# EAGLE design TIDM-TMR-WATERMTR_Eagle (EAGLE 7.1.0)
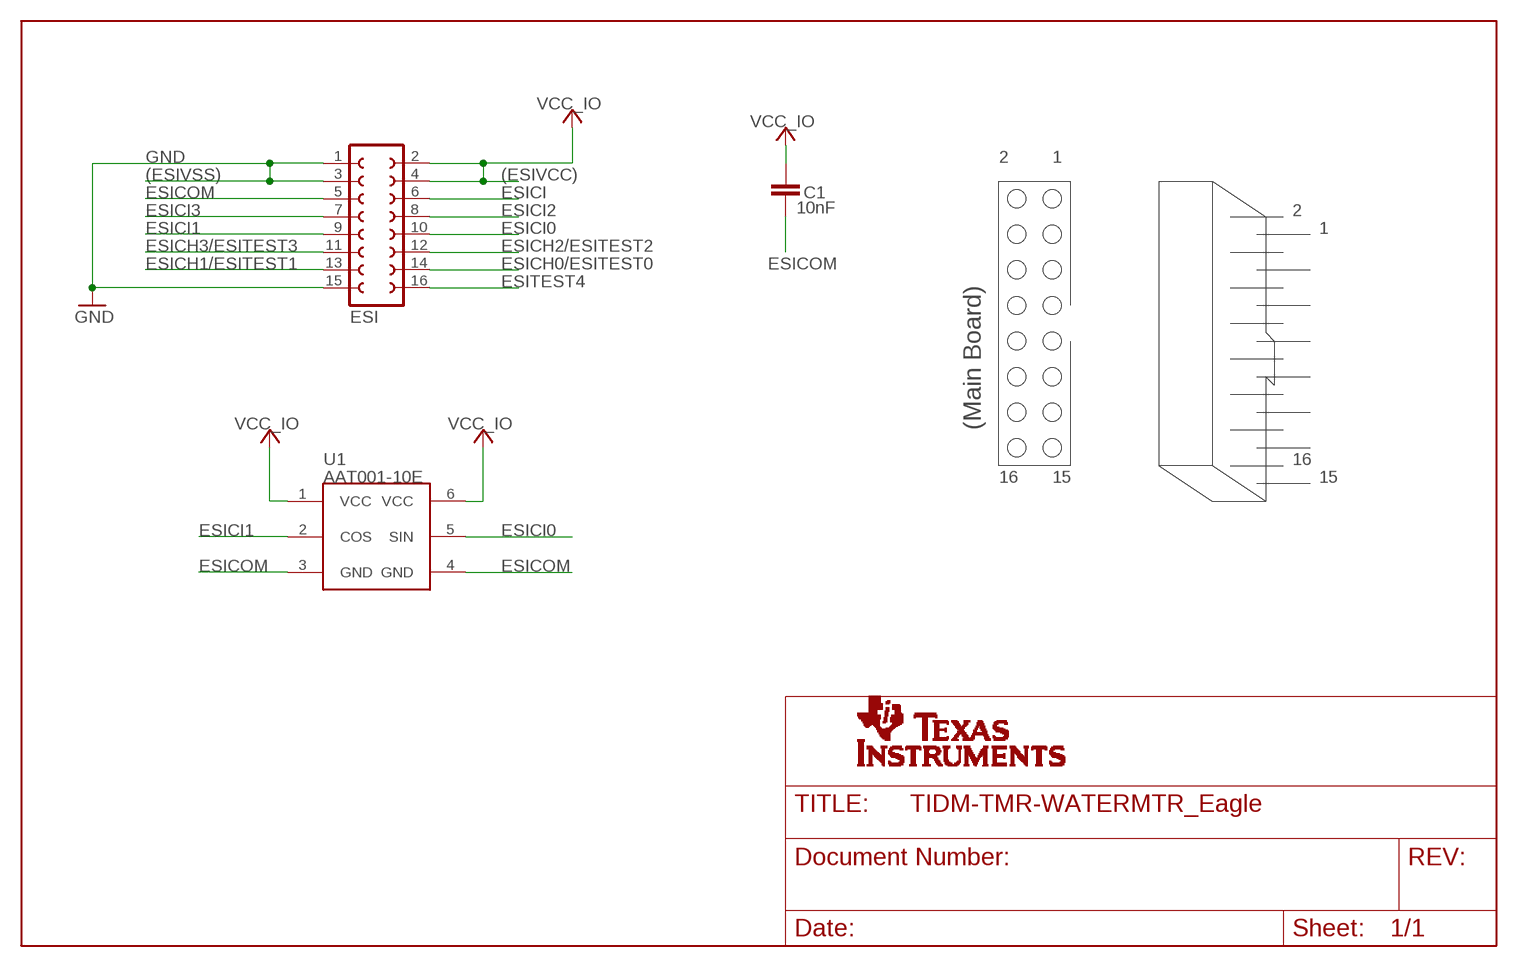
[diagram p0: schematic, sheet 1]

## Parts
C1  10nF  C-EUC0402K  [C0402K]
ESI  FE08-2  [FE08-2]
U1  AAT001-10E  [TDFN6-2.5X2.5MM]
U$1  TI-LOGO-SMALL  [TI-LOGO-4]

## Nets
ESICH0/ESITEST0: ESI.14
ESICH1/ESITEST1: ESI.13
ESICH2/ESITEST2: ESI.12
ESICH3/ESITEST3: ESI.11
ESICI: ESI.6
ESICI0: ESI.10 U1.5(SIN)
ESICI1: ESI.9 U1.2(COS)
ESICI2: ESI.8
ESICI3: ESI.7
ESICOM: C1.2 ESI.5 U1.3(GND) U1.4(GND)
ESITEST4: ESI.16
GND: ESI.1 ESI.3 ESI.15
VCC_IO: C1.1 ESI.2 ESI.4 U1.1(VCC) U1.6(VCC)

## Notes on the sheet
- 2 | 1
- (ESIVSS) | (ESIVCC)
- 2
- 1
- (Main Board)
- 16
- 16 | 15 | 15

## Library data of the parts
C1 = rcl:C-EU: CAPACITOR, European symbol
ESI = con-lsta:FE08-2: FEMALE HEADER; OC_FARNELL: unknown; OC_NEWARK: unknown
U1 = GMR Sensor:AAT001-10E
U$1 = texas-logo:TI-LOGO: Full TI logo

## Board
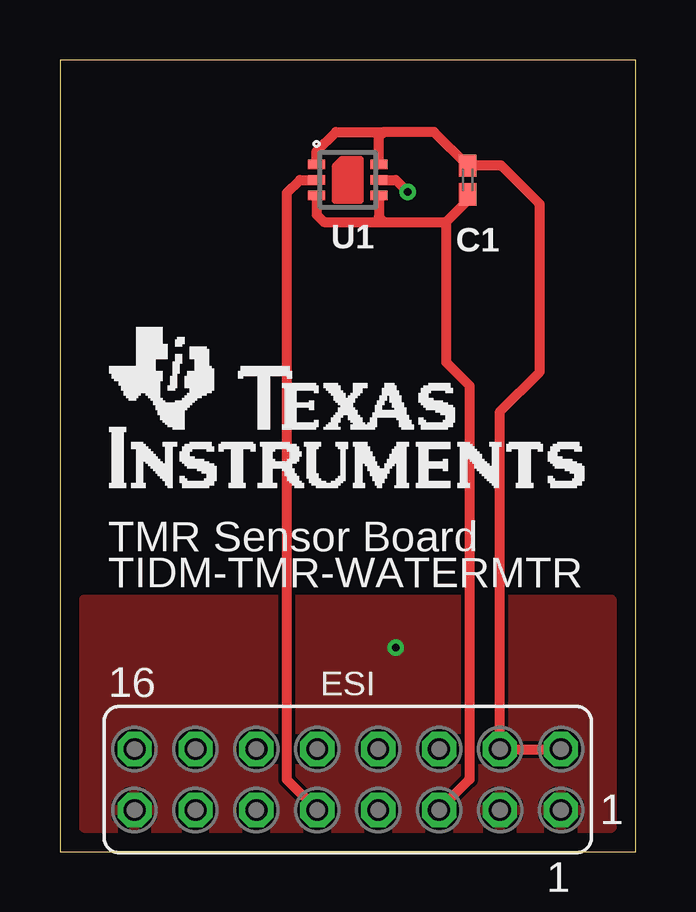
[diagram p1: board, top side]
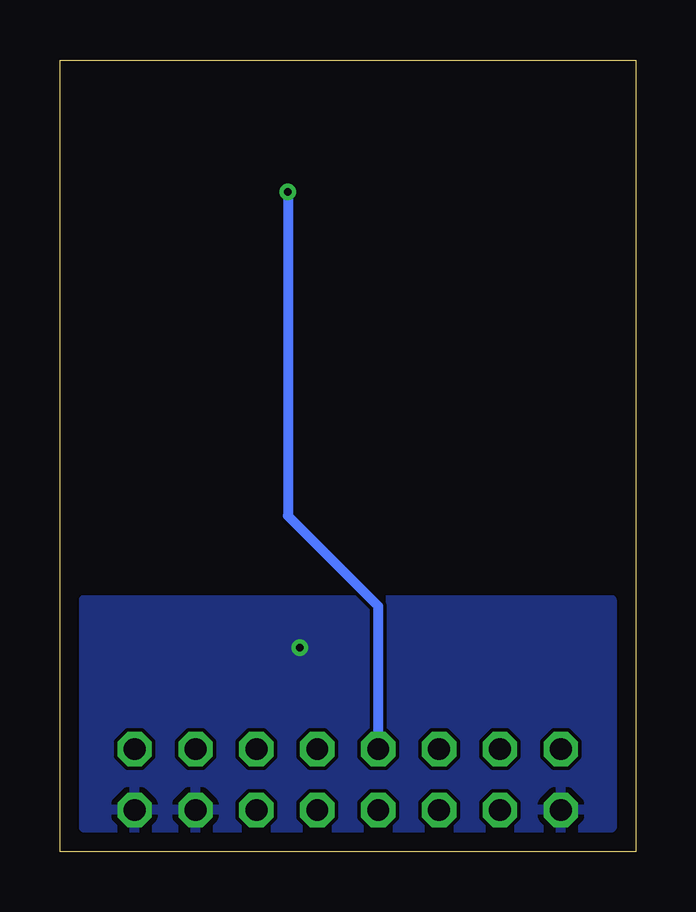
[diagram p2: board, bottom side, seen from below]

Size 24 x 33 mm. Coordinates in mm from the lower left corner, seen from the top.
Outline: 24,0 24,33 0,33 0,0 24,0
Copper layers (1*16): Top 0.035mm / dielectric 1.5mm / Bottom 0.035mm
Design rules "default *": minimum track width 10mil, minimum drill 0.3mm, track to track 6mil, track to pad 6mil, pad to pad 6mil, via to via 6mil, smd to smd 6mil, copper to edge 20mil, drill to drill 8mil, minimum pad ring 10mil, minimum via ring 8mil, stop-mask expansion 4mil, vias tented up to drill 100mil, thermal gap 10mil

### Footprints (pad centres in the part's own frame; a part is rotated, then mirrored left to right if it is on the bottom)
C0402K = smd 0.925 x 0.74: 1 -0.6,0; 2 0.6,0
FE08-2 = drill 0.914 octagon: 1 -8.89,1.27; 2 -8.89,-1.27; 3 -6.35,1.27; 4 -6.35,-1.27; 5 -3.81,1.27; 6 -3.81,-1.27; 7 -1.27,1.27; 8 -1.27,-1.27; 9 1.27,1.27; 10 1.27,-1.27; 11 3.81,1.27; 12 3.81,-1.27; 13 6.35,1.27; 14 6.35,-1.27; 15 8.89,1.27; 16 8.89,-1.27
TDFN6-2.5X2.5MM = smd 0.7 x 0.4: 1 -1.3,0.65; 2 -1.3,0; 3 -1.3,-0.65; 4 1.3,-0.65; 5 1.3,0; 6 1.3,0.65

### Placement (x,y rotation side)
C1  17,28 270 top
ESI  12,3 180 top
U1  12,28 0 top
U$1  2,15 0 top

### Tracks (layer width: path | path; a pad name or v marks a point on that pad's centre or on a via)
ESICI0  (via drill 0.3)
  Top 0.406: U1.5 14,28 v14.5,27.5
  Bottom 0.406: v14.5,27.5 14.5,14 10.73,10.23 ESI.10
ESICI1
  Top 0.406: ESI.9 9.46,3 9.46,27.46 10,28 U1.2
ESICOM
  Top 0.406: U1.3 10.7,26.55 11,26.25 13.5,26.25 | 13.5,26.25 16.1,26.25 | U1.4 13.3,26.45 13.5,26.25 | 16.1,26.25 16.1,20.4 17.08,19.42 17.08,3 ESI.5 | 16.1,26.25 17,27.15 C1.2
GND  (via drill 0.3)
  other vias: 14,8.5
  pour Bottom: 1,10.5 1,1 23,1 23,10.5
  pour Top: 1,10.5 1,1 23,1 23,10.5
VCC_IO
  Top 0.406: U1.1 10.7,29.2 11.5,30 13.5,30 | U1.6 13.3,29.8 13.5,30 | ESI.2 ESI.4 18.35,18.35 20,20 20,27 18.4,28.6 C1.1 15.6,30 13.5,30

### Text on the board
tPlace: TMR Sensor Board | TIDM-TMR-WATERMTR | 1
